|   This file is an IBIS representation of the   |
|   Integrated Device Technology Inc   |
|   IDT8V89317   |
|   Ethernet PLL for Industrial Automation and Power Systems   |
[IBIS Ver]   4.1
[File name]   8v89317.ibs
[File Rev]   1.3
|Rev 1.3,  Apr 14, 2014
|Created separate RLC package for non-Power signals
|Rev 1.2, 28 May 2013
|Corrected Pin Name H6,K7,L5,L6 from VDDA0 to VSSA0
|Updated differential LVPECL output driver model
|rev 1.1, May 15, 2013
|Updated RLC data
|rev 1.0, May 7, 2013
|Original model with place holder for RLC data.
[Notes]
The RLC values, including the power pins, have a max of >35pF capacitance. Some
simulators may use this value for a Min corner simulation of output signals, which
leads to incorrect results.  A separate Component was created to include only the
non-Power RLC values for these cases.  Use "IDT8V89317-BGA196-NonPowerRLC" to simulate
switching signals.
[Date]   14 Apr 2014
[Source]   Originated at Integrated Device Technology, Inc.
[Disclaimer]
IDT hereby grants the user of this IBIS model a non-exclusive,
nontransferable license to use this IBIS model under the following terms.
Before using this IBIS model, the user should read this license.
If the user does not accept these terms,  the IBIS model should be
returned to IDT within 30 days.
   The user is granted this license only to use the IBIS model and
is not granted rights to sell, load, rent, lease or license the IBIS
model in whole or in part, or in modified form to anyone other than
user. User may modify the IBIS model to suit its specific
applications but rights to derivative works and such modifications
shall belong to IDT.
   This IBIS model is provided on an AS IS basis and IDT makes
absolutely no warranty with respect to the information contained
herein. IDT DISCLAIMS AND CUSTOMER WAIVES ALL WARRANTIES, EXPRESS
OR IMPLIED, INCLUDING WARRANTIES OF MERCHANTABILITY OR FITNESS FOR
A PARTICULAR PURPOSE. The entire risk as to quality and performance
is with the Customer. ACCORDINGLY, IN NO EVENT SHALL THE COMPANY BE
LIABLE FOR ANY DAMAGES, WHETHER IN CONTRACT OR TORT,INCLUDING ANY
LOST PROFITS OR OTHER INCIDENTAL, CONSEQUENTIAL, EXEMPLARY, OR
PUNITIVE DAMAGES ARISING OUT OF THE USE OR APPLICATION OF THE IBIS
model provided in this package. Further, IDT reserves the right to
make changes without notice to any product herein to improve
reliability, function, or design. IDT does not convey any license
under patent rights or any other intellectual property rights,
including those of third parties.
   IDT is not obligated to provide maintenance or support
for the licensed IBIS model.
[Copyright]   Copyright 2013 by IDT Inc.
[Component]   IDT8V89317-BGA196-NonPowerRLC
[Manufacturer] Integrated Device Technology, Inc.
[Package]
|BGA 196
|lead + wire   typ   min   max
R_pkg   0.222   0.0515674   0.628939
L_pkg   3.206nH   0.886nH   9.061nH
C_pkg   1.171pF   0.497pF   3.985pF
[Pin]   signal_name   model_name   R_pin   L_pin   C_pin
A1   APLL1_LF0   NC   0.334348   4.73633nH   1.50284pF
A2   VDDA   POWER   0.08402   1.24995nH   4.93195pF
A3   IC1   NC
A4   CAP1   NC
A5   IN_APLL1_NEG INDIFF01N_PDPU100K  0.340484   5.61005nH   1.29913pF
A6   IC1   NC
A7   IC1   NC
A8   TDI   PDUSDGZ   0.142959   2.16014nH   0.622557pF
A9   VC0   NC
A10   IC2   NC
A11   OSCI   NC
A12   TMS   PDUSDGZ   0.158506   2.27988nH   0.666767pF
A13   VC4   NC
A14   TRST   PDDSDGZ   0.164723   2.1921nH   0.675437pF
B1   APLL1_LF1   NC   0.278229   4.23554nH   1.78426pF
B2   VSSA   GND
B3   IC1   NC
B4   VSSA0   GND
B5   IN_APPL1_POS INDIFF01P_PDPU100K  0.310265   5.16569nH   1.20038pF
B6   IC1   NC
B7   IC1   NC
B8   TDO   PDT02DGZ   0.176917   2.41141nH   0.655527pF
B9   VSSA0   GND
B10   TCK   PDDSDGZ   0.221025   2.95269nH   0.841653pF
B11   VSSA   GND
B12   VDDA   POWER   0.0753102   1.19036nH   3.15432pF
B13   VSSD0   GND
B14   VDDD0   POWER   0.0371692   0.689269nH   5.71412pF
C1   ISET_APLL1   NC   0.254219   3.28566nH   1.08299pF
C2   VDDA   POWER   0.08402   1.24995nH   4.93195pF
C3   NC   NC
C4   CAP2   NC
C5   IC1   NC
C6   IC1   NC
C7   VDDDO   POWER   0.0515674   0.886249nH   3.58412pF
C8   VSSDO   GND
C9   VDDA   POWER   0.0753102   1.19036nH   3.15432pF
C10   VSSA   GND
C11   VDDA   POWER   0.0753102   1.19036nH   3.15432pF
C12   VDDA   POWER   0.08402   1.24995nH   4.93195pF
C13   INT_REQ   PDT02DGZ   0.133505   1.88864nH   0.636295pF
C14   IC1   NC
D1   VSSA   GND
D2   VSSA0   GND
D3   CAP3   NC
D4   VSSA   GND
D5   VDDA   POWER   0.0753102   1.19036nH   3.15432pF
D6   IC1   NC
D7   VSSD   GND
D8   VDDD   POWER   0.0733794   1.32964nH   1.20295pF
D9   IC1   NC
D10   VDDA   POWER   0.0753102   1.19036nH   3.15432pF
D11   VSSA   GND
D12   VDDA   POWER   0.0753102   1.19036nH   3.15432pF
D13   IC1   NC
D14   IC1   NC
E1   XTAL1_IN   NC   0.334819   4.75366nH   1.5807pF
E2   XTAL1_OUT   NC   0.284387   4.11262nH   1.33295pF
E3   VSSA   GND
E4   VSSA0   GND
E5   VSSA   GND
E6   IC3   NC
E7   VSSD   GND
E8   VDDD   POWER   0.0733794   1.32964nH   1.20295pF
E9   IC1   NC
E10   VSSA   GND
E11   VDDA   POWER   0.0753102   1.19036nH   3.15432pF
E12   VSSA   GND
E13   IC1   NC
E14   IC1   NC
F1   VDDD   POWER   0.0186506   0.320268nH   17.9991pF
F2   VSSD   GND
F3   VSSA0   GND
F4   VSSA   GND
F5   VDDA   POWER   0.0753102   1.19036nH   3.15432pF
F6   VSSA0   GND
F7   VSSD   GND
F8   VDDD   POWER   0.0733794   1.32964nH   1.20295pF
F9   VSSD   GND
F10   VDDD   POWER   0.0733794   1.32964nH   1.20295pF
F11   IC1   NC
F12   VDDDO   POWER   0.094203   1.48743nH   2.89182pF
F13   OUT4   PDO04CDG   0.155809   2.11446nH   0.660969pF
F14   VSSDO   GND
G1   VSSD   GND
G2   VDDD   POWER   0.0276409   0.422404nH   35.2531pF
G3   VSSA0   GND
G4   VSSA0   GND
G5   VSSA0   GND
G6   VSSD   GND
G7   VDDD   POWER   0.068222   0.90552nH   5.32678pF
G8   IC1   NC
G9   VDDD   POWER   0.0371692   0.689269nH   5.71412pF
G10   VSSD   GND
G11   IC1   GND
G12   IC1   GND
G13   IC1   GND
G14   IC1   GND
H1   VDDA0   POWER   0.068222   0.90552nH   5.32678pF
H2   VSSA0   GND
H3   VDDAO   POWER   0.08402   1.24995nH   4.93195pF
H4   VSSA0   GND
H5   VSSAO   GND
H6   VDDAO   GND
H7   VSSD   GND
H8   VDDD   POWER   0.068222   0.90552nH   5.32678pF
H9   VSSD   GND
H10   VDDD   POWER   0.068222   0.90552nH   5.32678pF
H11   IC1   NC
H12   IC1   NC
H13   RST   PDUSDGZ   0.83377   12.1862nH   3.88243pF
H14   IN1   ami_rx   0.196725   2.76061nH   0.726838pF
J1   OUT1_NEG   PECL_LVDS04   0.252954   3.53133nH   0.730914pF
J2   OUT1_POS   PECL_LVDS04   0.246367   3.34809nH   0.699321pF
J3   VDDAO   POWER   0.08402   1.24995nH   4.93195pF
J4   VSSAO   GND
J5   VDDAO   POWER   0.08402   1.24995nH   4.93195pF
J6   VSSAO   GND
J7   VDDAO   POWER   0.08402   1.24995nH   4.93195pF
J8   VSSAO   GND
J9   VSSA   GND
J10   VDDA   POWER   0.0753102   1.19036nH   3.15432pF
J11   DPLL_LOCK   PDT02DGZ   0.131397   2.24181nH   0.729437pF
J12   IC1   NC
J13   IN2   ami_rx   0.160825   2.31934nH   0.67745pF
J14   IN3   ami_rx   0.362282   5.2171nH   1.60392pF
K1   VSSAO   GND
K2   VSSAO   GND
K3   VSSAO   GND
K4   VDDAO   POWER   0.08402   1.24995nH   4.93195pF
K5   VSSAO   GND
K6   VDDAO   POWER   0.08402   1.24995nH   4.93195pF
K7   VDDAO   GND
K8   VSSD   GND
K9   VDDD   POWER   0.068222   0.90552nH   5.32678pF
K10   VSSAO   GND
K11   IC1   NC
K12   IC1   NC
K13   I2C_SCL   PDDSDGZ   0.601196   9.0618nH   2.89322pF
K14   I2C_SDA   PDD02SDGZ   0.283464   4.89492nH   3.98528pF
L1   OUT2_NEG   PECL_LVDS04   0.172003   2.36707nH   0.531051pF
L2   OUT2_POS   PECL_LVDS04   0.158041   2.1493nH   0.497244pF
L3   VDDA0   POWER   0.08402   1.24995nH   4.93195pF
L4   VSSAO   GND
L5   VDDAO   GND
L6   VDDAO   GND
L7   VSSAO   GND
L8   I2C_AD1   PDUSDGZ   0.628939   7.3282nH   3.17476pF
L9   I2C_AD2   PDUSDGZ   0.579908   7.18207nH   2.82964pF
L10   CAP4   NC
L11   VSSA   GND
L12   CAP5   NC
L13   VSSA   GND
L14   CAP6   NC
M1   VDDAO   POWER   0.08402   1.24995nH   4.93195pF
M2   VSSAO   GND
M3   VSSAO   GND
M4   VSSADO   GND
M5   VDDAO   POWER   0.08402   1.24995nH   4.93195pF
M6   VSSAO   GND
M7   VDDAO   POWER   0.08402   1.24995nH   4.93195pF
M8   VSSAO   GND
M9   VSSAO   GND
M10   VSSAO   GND
M11   VSSAO   GND
M12   NC   NC
M13   NC   NC
M14   NC   NC
N1   VSSAO   GND
N2   OUT3_POS   PECL_LVDS04   0.134275   1.83601nH   0.60374pF
N3   VSSAO   GND
N4   IC1   NC
N5   VSSAO   GND
N6   IN_APLL2_POS INDIFF01P_PDPU100K  0.264444   3.49073nH   0.768733pF
N7   IC2   NC
N8   I2C   NC
N9   VSSA   GND
N10   XTAL2_OUT   NC   0.180966   2.37539nH   0.741578pF
N11   VSSA   GND
N12   APLL2_LF1   NC   0.159345   2.18796nH   1.07785pF
N13   VSSAO   GND
N14   VSSA   GND
P1   VDDAO   POWER   0.08402   1.24995nH   4.93195pF
P2   OUT3_NEG   PECL_LVDS04   0.226993   3.03703nH   0.665671pF
P3   VSSAO   GND
P4   IC1   NC
P5   VDDAO   POWER   0.068222   0.90552nH   5.32678pF
P6   IN_APLL2_NEG INDIFF01N_PDPU100K  0.340484   5.61005nH   1.29913pF
P7   IC2   NC
P8   IC2   NC
P9   VDDA   POWER   0.0753102   1.19036nH   3.15432pF
P10   XTAL2_IN   NC   0.163448   2.22776nH   0.674849pF
P11   VDDA   POWER   0.08402   1.24995nH   4.93195pF
P12   APLL2_LFO   NC   0.214835   2.96596nH   1.55911pF
P13   ISTE_APLL2   NC   0.256779   3.60749nH   1.80531pF
P14   VDDA   POWER   0.0753102   1.19036nH   3.15432pF
[Diff Pin]   inv_pin vdiff   tdelay_typ   tdelay_min   tdelay_max
|Inputs
B5   A5   150mV   NA   NA   NA
N6   P6   150mV   NA   NA   NA
|Outputs
J2   J1   NA   0   0   0
L2   L1   NA   0   0   0
N2   P2   NA   0   0   0
[Component]   IDT82V3910-BGA196-PowerRLC
[Manufacturer] Integrated Device Technology, Inc.
[Package]
|BGA 196
|lead + wire   typ   min   max
R_pkg   0.3069   0.01865   1.0645
L_pkg   4.3859nF   0.32027nF   16.561nF
C_pkg   2.7933pF   0.49724pF   35.307pF
[Pin]   signal_name   model_name   R_pin   L_pin   C_pin
A1   APLL1_LF0   NC   0.334348   4.73633nH   1.50284pF
A2   VDDA   POWER   0.08402   1.24995nH   4.93195pF
A3   IC1   NC
A4   CAP1   NC
A5   IN_APLL1_NEG INDIFF01N_PDPU100K  0.340484   5.61005nH   1.29913pF
A6   IC1   NC
A7   IC1   NC
A8   TDI   PDUSDGZ   0.142959   2.16014nH   0.622557pF
A9   VC0   NC
A10   IC2   NC
A11   OSCI   NC
A12   TMS   PDUSDGZ   0.158506   2.27988nH   0.666767pF
A13   VC4   NC
A14   TRST   PDDSDGZ   0.164723   2.1921nH   0.675437pF
B1   APLL1_LF1   NC   0.278229   4.23554nH   1.78426pF
B2   VSSA   GND
B3   IC1   NC
B4   VSSA0   GND
B5   IN_APPL1_POS INDIFF01P_PDPU100K  0.310265   5.16569nH   1.20038pF
B6   IC1   NC
B7   IC1   NC
B8   TDO   PDT02DGZ   0.176917   2.41141nH   0.655527pF
B9   VSSA0   GND
B10   TCK   PDDSDGZ   0.221025   2.95269nH   0.841653pF
B11   VSSA   GND
B12   VDDA   POWER   0.0753102   1.19036nH   3.15432pF
B13   VSSD0   GND
B14   VDDD0   POWER   0.0371692   0.689269nH   5.71412pF
C1   ISET_APLL1   NC   0.254219   3.28566nH   1.08299pF
C2   VDDA   POWER   0.08402   1.24995nH   4.93195pF
C3   NC   NC
C4   CAP2   NC
C5   IC1   NC
C6   IC1   NC
C7   VDDDO   POWER   0.0515674   0.886249nH   3.58412pF
C8   VSSDO   GND
C9   VDDA   POWER   0.0753102   1.19036nH   3.15432pF
C10   VSSA   GND
C11   VDDA   POWER   0.0753102   1.19036nH   3.15432pF
C12   VDDA   POWER   0.08402   1.24995nH   4.93195pF
C13   INT_REQ   PDT02DGZ   0.133505   1.88864nH   0.636295pF
C14   IC1   NC
D1   VSSA   GND
D2   VSSA0   GND
D3   CAP3   NC
D4   VSSA   GND
D5   VDDA   POWER   0.0753102   1.19036nH   3.15432pF
D6   IC1   NC
D7   VSSD   GND
D8   VDDD   POWER   0.0733794   1.32964nH   1.20295pF
D9   IC1   NC
D10   VDDA   POWER   0.0753102   1.19036nH   3.15432pF
D11   VSSA   GND
D12   VDDA   POWER   0.0753102   1.19036nH   3.15432pF
D13   IC1   NC
D14   IC1   NC
E1   XTAL1_IN   NC   0.334819   4.75366nH   1.5807pF
E2   XTAL1_OUT   NC   0.284387   4.11262nH   1.33295pF
E3   VSSA   GND
E4   VSSA0   GND
E5   VSSA   GND
E6   IC3   NC
E7   VSSD   GND
E8   VDDD   POWER   0.0733794   1.32964nH   1.20295pF
E9   IC1   NC
E10   VSSA   GND
E11   VDDA   POWER   0.0753102   1.19036nH   3.15432pF
E12   VSSA   GND
E13   IC1   NC
E14   IC1   NC
F1   VDDD   POWER   0.0186506   0.320268nH   17.9991pF
F2   VSSD   GND
F3   VSSA0   GND
F4   VSSA   GND
F5   VDDA   POWER   0.0753102   1.19036nH   3.15432pF
F6   VSSA0   GND
F7   VSSD   GND
F8   VDDD   POWER   0.0733794   1.32964nH   1.20295pF
F9   VSSD   GND
F10   VDDD   POWER   0.0733794   1.32964nH   1.20295pF
F11   IC1   NC
F12   VDDDO   POWER   0.094203   1.48743nH   2.89182pF
F13   OUT4   PDO04CDG   0.155809   2.11446nH   0.660969pF
F14   VSSDO   GND
G1   VSSD   GND
G2   VDDD   POWER   0.0276409   0.422404nH   35.2531pF
G3   VSSA0   GND
G4   VSSA0   GND
G5   VSSA0   GND
G6   VSSD   GND
G7   VDDD   POWER   0.068222   0.90552nH   5.32678pF
G8   IC1   NC
G9   VDDD   POWER   0.0371692   0.689269nH   5.71412pF
G10   VSSD   GND
G11   IC1   GND
G12   IC1   GND
G13   IC1   GND
G14   IC1   GND
H1   VDDA0   POWER   0.068222   0.90552nH   5.32678pF
H2   VSSA0   GND
H3   VDDAO   POWER   0.08402   1.24995nH   4.93195pF
H4   VSSA0   GND
H5   VSSAO   GND
H6   VDDAO   GND
H7   VSSD   GND
H8   VDDD   POWER   0.068222   0.90552nH   5.32678pF
H9   VSSD   GND
H10   VDDD   POWER   0.068222   0.90552nH   5.32678pF
H11   IC1   NC
H12   IC1   NC
H13   RST   PDUSDGZ   0.83377   12.1862nH   3.88243pF
H14   IN1   ami_rx   0.196725   2.76061nH   0.726838pF
J1   OUT1_NEG   PECL_LVDS04   0.252954   3.53133nH   0.730914pF
J2   OUT1_POS   PECL_LVDS04   0.246367   3.34809nH   0.699321pF
J3   VDDAO   POWER   0.08402   1.24995nH   4.93195pF
J4   VSSAO   GND
J5   VDDAO   POWER   0.08402   1.24995nH   4.93195pF
J6   VSSAO   GND
J7   VDDAO   POWER   0.08402   1.24995nH   4.93195pF
J8   VSSAO   GND
J9   VSSA   GND
J10   VDDA   POWER   0.0753102   1.19036nH   3.15432pF
J11   DPLL_LOCK   PDT02DGZ   0.131397   2.24181nH   0.729437pF
J12   IC1   NC
J13   IN2   ami_rx   0.160825   2.31934nH   0.67745pF
J14   IN3   ami_rx   0.362282   5.2171nH   1.60392pF
K1   VSSAO   GND
K2   VSSAO   GND
K3   VSSAO   GND
K4   VDDAO   POWER   0.08402   1.24995nH   4.93195pF
K5   VSSAO   GND
K6   VDDAO   POWER   0.08402   1.24995nH   4.93195pF
K7   VDDAO   GND
K8   VSSD   GND
K9   VDDD   POWER   0.068222   0.90552nH   5.32678pF
K10   VSSAO   GND
K11   IC1   NC
K12   IC1   NC
K13   I2C_SCL   PDDSDGZ   0.601196   9.0618nH   2.89322pF
K14   I2C_SDA   PDD02SDGZ   0.283464   4.89492nH   3.98528pF
L1   OUT2_NEG   PECL_LVDS04   0.172003   2.36707nH   0.531051pF
L2   OUT2_POS   PECL_LVDS04   0.158041   2.1493nH   0.497244pF
L3   VDDA0   POWER   0.08402   1.24995nH   4.93195pF
L4   VSSAO   GND
L5   VDDAO   GND
L6   VDDAO   GND
L7   VSSAO   GND
L8   I2C_AD1   PDUSDGZ   0.628939   7.3282nH   3.17476pF
L9   I2C_AD2   PDUSDGZ   0.579908   7.18207nH   2.82964pF
L10   CAP4   NC
L11   VSSA   GND
L12   CAP5   NC
L13   VSSA   GND
L14   CAP6   NC
M1   VDDAO   POWER   0.08402   1.24995nH   4.93195pF
M2   VSSAO   GND
M3   VSSAO   GND
M4   VSSADO   GND
M5   VDDAO   POWER   0.08402   1.24995nH   4.93195pF
M6   VSSAO   GND
M7   VDDAO   POWER   0.08402   1.24995nH   4.93195pF
M8   VSSAO   GND
M9   VSSAO   GND
M10   VSSAO   GND
M11   VSSAO   GND
M12   NC   NC
M13   NC   NC
M14   NC   NC
N1   VSSAO   GND
N2   OUT3_POS   PECL_LVDS04   0.134275   1.83601nH   0.60374pF
N3   VSSAO   GND
N4   IC1   NC
N5   VSSAO   GND
N6   IN_APLL2_POS INDIFF01P_PDPU100K  0.264444   3.49073nH   0.768733pF
N7   IC2   NC
N8   I2C   NC
N9   VSSA   GND
N10   XTAL2_OUT   NC   0.180966   2.37539nH   0.741578pF
N11   VSSA   GND
N12   APLL2_LF1   NC   0.159345   2.18796nH   1.07785pF
N13   VSSAO   GND
N14   VSSA   GND
P1   VDDAO   POWER   0.08402   1.24995nH   4.93195pF
P2   OUT3_NEG   PECL_LVDS04   0.226993   3.03703nH   0.665671pF
P3   VSSAO   GND
P4   IC1   NC
P5   VDDAO   POWER   0.068222   0.90552nH   5.32678pF
P6   IN_APLL2_NEG INDIFF01N_PDPU100K  0.340484   5.61005nH   1.29913pF
P7   IC2   NC
P8   IC2   NC
P9   VDDA   POWER   0.0753102   1.19036nH   3.15432pF
P10   XTAL2_IN   NC   0.163448   2.22776nH   0.674849pF
P11   VDDA   POWER   0.08402   1.24995nH   4.93195pF
P12   APLL2_LFO   NC   0.214835   2.96596nH   1.55911pF
P13   ISTE_APLL2   NC   0.256779   3.60749nH   1.80531pF
P14   VDDA   POWER   0.0753102   1.19036nH   3.15432pF
[Diff Pin]   inv_pin vdiff   tdelay_typ   tdelay_min   tdelay_max
|Inputs
B5   A5   150mV   NA   NA   NA
N6   P6   150mV   NA   NA   NA
|Outputs
J2   J1   NA   0   0   0
L2   L1   NA   0   0   0
N2   P2   NA   0   0   0
| Models and submodels in the file (9): PECL_LVDS04 (Output_ECL), PDDSDGZ (Input), PDUSDGZ (Input), ami_rx (Input), PDT02DGZ (3-state), PDD02SDGZ (I/O), PDO04CDG (Output), INDIFF01P_PDPU100K (Input), INDIFF01N_PDPU100K (Input)
